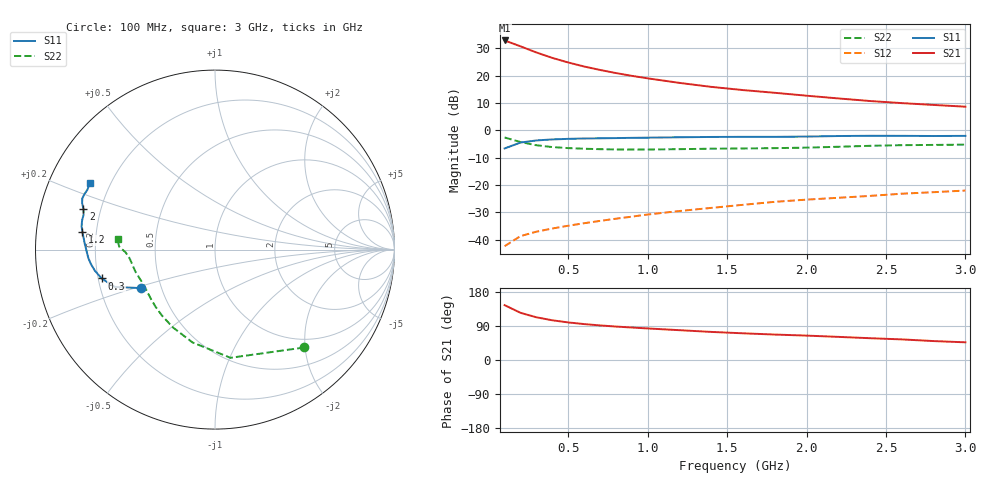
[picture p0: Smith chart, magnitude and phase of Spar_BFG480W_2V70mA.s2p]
! Filename: 270BFG480.001
! Title: BFG480W
! Bias: Vce=2V; Ic=70mA
! Company: NXP Semiconductors NL
! User: Quality&Reliability T&D
! Measure time: 10 Nov 1999 / 11:54:25
#  MHz  S  MA  R 50
! Freq  S11  S21  S12  S22  :
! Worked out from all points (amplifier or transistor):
!   20 points, 100 MHz to 3 GHz, reference 50 ohm
!   highest |S21| = 32.9 dB at 100 MHz (marker M1)
!   |S21| within 3 dB of that: start of sweep to 238 MHz
!   unconditionally stable (mu >= 1): 767.6 MHz to end of sweep
!   at 400 MHz: K = 0.77, MSG = 31.2 dB, |S12| = -36.0 dB
!   at 1.2 GHz: K = 1.08, MAG = 21.7 dB, |S12| = -29.6 dB
!   at 3 GHz: K = 1.10, MAG = 13.4 dB, |S12| = -22.1 dB
!   S11 on the Smith chart (normalised r, x): 100 MHz: 0.38, -0.21; 300 MHz: 0.21, -0.12; 1.2 GHz: 0.15, +0.06; 2 GHz: 0.13, +0.15; 3 GHz: 0.12, +0.24
100  0.4649 -152.5  44.1 144.8  0.007553 67.1  0.7379 -47.6
200  0.5959 -159.6  34.44 124.5  0.01154 57.2  0.609 -81.9
300  0.6515 -165.7  26.59 112.7  0.01392 55.3  0.532 -103.7
400  0.6799 -170.1  21.13 104.8  0.01591 56.4  0.4928 -118.4
500  0.6962 -173.4  17.43 99.2  0.01786 58.2  0.4717 -128.7
600  0.7073 -176.2  14.72 94.8  0.01986 60.1  0.4592 -136.2
700  0.7133 -178.5  12.73 91.3  0.02191 62.2  0.4508 -142.0
800  0.7193 179.4  11.17 88.3  0.02403 64.0  0.4459 -146.7
900  0.7265 177.4  9.926 85.7  0.02621 65.8  0.4436 -150.7
1000  0.7322 175.6  8.933 83.3  0.0287 67.0  0.4441 -154.3
1200  0.7448 172.5  7.375 78.7  0.03323 68.8  0.4509 -160.0
1400  0.7544 170.1  6.236 74.1  0.03791 69.9  0.4597 -164.3
1600  0.758 167.7  5.446 70.4  0.04319 70.8  0.4645 -167.7
1800  0.7577 165.1  4.855 67.1  0.04896 71.5  0.4708 -171.1
2000  0.767 162.9  4.297 64.4  0.05372 72.4  0.4812 -175.1
2200  0.7846 160.7  3.831 61.0  0.05808 72.3  0.4989 -178.3
2400  0.7924 158.9  3.432 57.5  0.06289 71.9  0.5194 179.7
2600  0.7907 157.1  3.142 54.4  0.06893 71.2  0.5336 178.3
2800  0.7853 154.8  2.91 49.9  0.07356 69.9  0.5394 176.4
3000  0.7895 152.2  2.704 46.6  0.07879 69.2  0.5458 173.6
